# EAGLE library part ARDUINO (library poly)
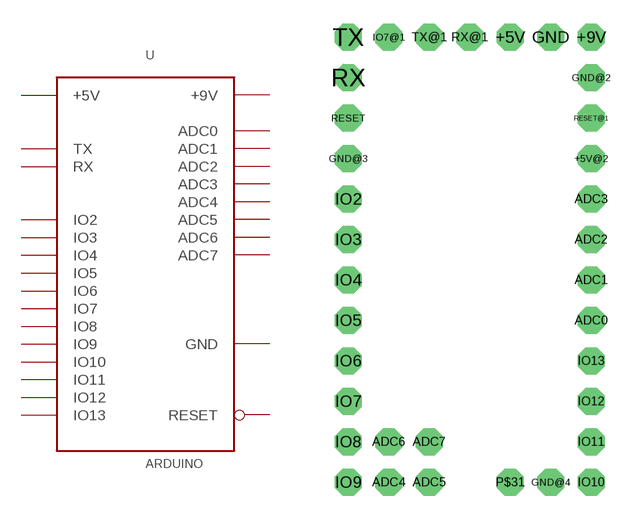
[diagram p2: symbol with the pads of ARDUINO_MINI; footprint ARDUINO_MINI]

Designator prefix -

## ARDUINO  [ARDUINO_MINI]
+5V  +5V  pwr
+5V@2  +5V  pwr
+9V  +9V  pwr
ADC0  ADC0  in
ADC1  ADC1  in
ADC2  ADC2  in
ADC3  ADC3  in
ADC4  ADC4  in
ADC5  ADC5  in
ADC6  ADC6  in
ADC7  ADC7  in
GND  GND  sup
GND@2  GND  sup
GND@3  GND  sup
GND@4  GND  sup
IO2  IO2
IO3  IO3
IO4  IO4
IO5  IO5
IO6  IO6
IO7  IO7
IO7@1  IO7
IO8  IO8
IO9  IO9
IO10  IO10
IO11  IO11
IO12  IO12
IO13  IO13
P$31  +5V  pwr
RESET  RESET
RESET@1  RESET
RX  RX  in
RX@1  RX  in
TX  TX  out
TX@1  TX  out

## Footprint ARDUINO_MINI (pad centres in mm)
drill 0.8 pad 1.676 octagon: +5V 11.43,29.21; +5V@2 16.51,21.59; +9V 16.51,29.21; ADC0 16.51,11.43; ADC1 16.51,13.97; ADC2 16.51,16.51; ADC3 16.51,19.05; ADC4 3.81,1.27; ADC5 6.35,1.27; ADC6 3.81,3.81; ADC7 6.35,3.81; GND 13.97,29.21; GND@2 16.51,26.67; GND@3 1.27,21.59; GND@4 13.97,1.27; IO2 1.27,19.05; IO3 1.27,16.51; IO4 1.27,13.97; IO5 1.27,11.43; IO6 1.27,8.89; IO7 1.27,6.35; IO7@1 3.81,29.21; IO8 1.27,3.81; IO9 1.27,1.27; IO10 16.51,1.27; IO11 16.51,3.81; IO12 16.51,6.35; IO13 16.51,8.89; P$31 11.43,1.27; RESET 1.27,24.13; RESET@1 16.51,24.13; RX 1.27,26.67; RX@1 8.89,29.21; TX 1.27,29.21; TX@1 6.35,29.21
